FUNCTION_BLOCK FB_DO_IED_LD1_LEDGGIO5_NamPlt EXTENDS FB_AcsiCommonDataClass
VAR_INPUT
	vendor: FB_AcsiDATypeVisString255 := (fc:=ACSI_FC_DC, bLinkResult:=THIS^.AddDataToContainer(ipData:=vendor));
	swRev: FB_AcsiDATypeVisString255 := (fc:=ACSI_FC_DC, bLinkResult:=THIS^.AddDataToContainer(ipData:=swRev));
	d: FB_AcsiDATypeVisString255 := (fc:=ACSI_FC_DC, bLinkResult:=THIS^.AddDataToContainer(ipData:=d));
END_VAR
VAR
END_VAR

END_FUNCTION_BLOCK
